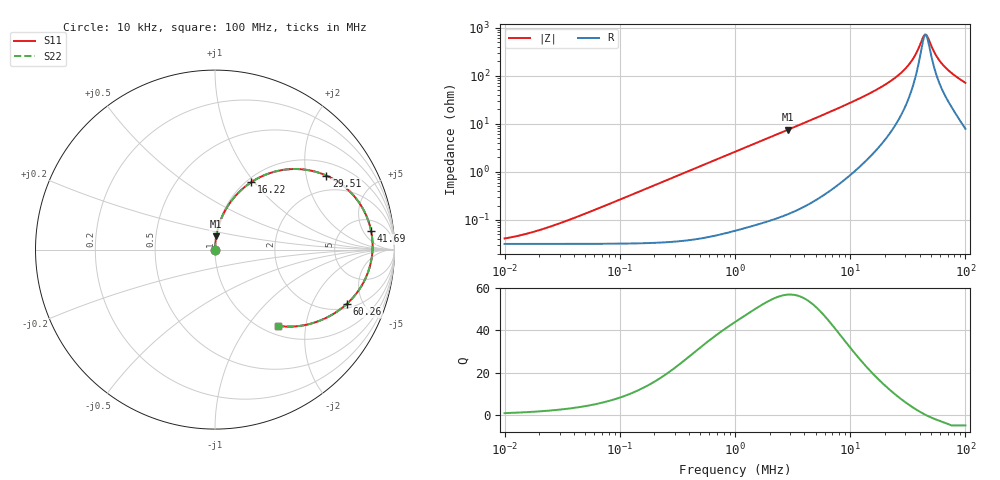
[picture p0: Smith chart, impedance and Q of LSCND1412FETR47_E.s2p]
! LSCND1412FETR47_E  S-PARAMETER MODEL  ( Standard Model )
! Model Generated by TAIYO YUDEN Corporation (http://www.ty-top.com)
! Version 1.0
! TAIYO YUDEN Control No. 231226
! Copyright(c) 2023 TAIYO YUDEN CO.,LTD. All Rights Reserved.
! Product Description (link to TY-COMPAS)
! https://ds.yuden.co.jp/TYCOMPAS/or/detail?pn=LSCND1412FETR47ME&u=M
! Products Name : Inductors
! Characteristics :
!  Inductance : 0.47 [uH] , SRF(min) : - [Hz] , DC Resistance(max) : 38 [mOhm]
!  Rated Current : Saturation  3.6 [A] (dL = 30 [%]), Temp Rise  3.4 [A] (dT = 40 [degC])
!  Case Size : 1.4 x 1.2 / 0.055 x 0.047 [mm/inch] , Thickness : 0.65 / 0.026 [mm/inch]
!  (Conditions: Temperature = 25 [degC] , DC Bias Current = 0 [A])
! External Node Assignments :
!  1  o---GGG---o  2
! GND o---------o GND
! Frequency Range : 10kHz  -  100MHz  [ 402 STEP ]
# MHz S RI R 50
! Freq[MHz].  S11 Real  S11 Imag  S21 Real  S21 Imag  S12 Real  S12 Imag  S22 Real  S22 Imag
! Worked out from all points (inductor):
!   401 points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, 10 kHz to 100 MHz, reference 50 ohm
!   read as one part in series: L = 418 nH near 37.15 kHz
!   highest Q = 56.8 at 2.884 MHz (marker M1), where L = 414 nH
!   self-resonance near 45.15 MHz
!   S11 on the Smith chart (normalised r, x): 10 kHz: 1.00, +0.00; 16.22 MHz: 1.05, +0.96; 29.51 MHz: 1.41, +2.62; 41.69 MHz: 8, +7; 60.26 MHz: 2.28, -3.74; 100 MHz: 1.16, -1.41
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0.01  0.000318 0.000263  0.9997 -0.000263  0.9997 -0.000263  0.000318 0.000263
0.019498  0.000318 0.000512  0.9997 -0.000512  0.9997 -0.000512  0.000318 0.000512
0.046774  0.00032 0.00123  0.9997 -0.00123  0.9997 -0.00123  0.00032 0.00123
0.218776  0.000371 0.00574  0.9996 -0.00574  0.9996 -0.00574  0.000371 0.00574
1  0.00128 0.0261  0.9987 -0.0261  0.9987 -0.0261  0.00128 0.0261
2.884032  0.0069 0.0745  0.9931 -0.0745  0.9931 -0.0745  0.0069 0.0745
4.677351  0.017 0.1201  0.983 -0.1201  0.983 -0.1201  0.017 0.1201
9.772372  0.0723 0.2441  0.9277 -0.2441  0.9277 -0.2441  0.0723 0.2441
16.2181  0.201 0.3749  0.799 -0.3749  0.799 -0.3749  0.201 0.3749
21.87762  0.3645 0.4415  0.6355 -0.4415  0.6355 -0.4415  0.3645 0.4415
25.70396  0.4922 0.4466  0.5078 -0.4466  0.5078 -0.4466  0.4922 0.4466
29.51209  0.6197 0.4128  0.3803 -0.4128  0.3803 -0.4128  0.6197 0.4128
35.48134  0.7842 0.287  0.2158 -0.287  0.2158 -0.287  0.7842 0.287
38.01894  0.8311 0.2147  0.1689 -0.2147  0.1689 -0.2147  0.8311 0.2147
41.68694  0.87 0.1029  0.13 -0.1029  0.13 -0.1029  0.87 0.1029
43.65158  0.8776 0.0435  0.1224 -0.0435  0.1224 -0.0435  0.8776 0.0435
45.70882  0.8768 -0.016  0.1232 0.016  0.1232 0.016  0.8768 -0.016
47.86301  0.8679 -0.0741  0.1321 0.0741  0.1321 0.0741  0.8679 -0.0741
54.95409  0.8011 -0.2261  0.1989 0.2261  0.1989 0.2261  0.8011 -0.2261
60.25596  0.7351 -0.3019  0.2649 0.3019  0.2649 0.3019  0.7351 -0.3019
74.13102  0.5698 -0.4012  0.4302 0.4012  0.4302 0.4012  0.5698 -0.4012
100  0.3503 -0.4246  0.6497 0.4246  0.6497 0.4246  0.3503 -0.4246
